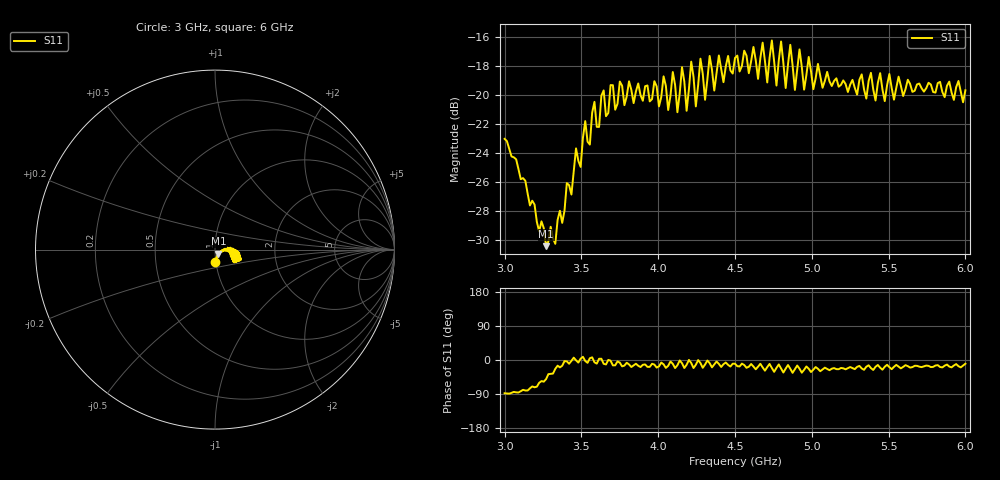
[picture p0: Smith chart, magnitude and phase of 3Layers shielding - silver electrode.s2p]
!  03/07/2025  15:49:02
! Ref Plane: 0.000 mm
# MHZ S MA R  50
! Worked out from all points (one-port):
!   201 points, 3 GHz to 6 GHz, reference 50 ohm
!   lowest |S11| = -30.4 dB at 3.27 GHz (marker M1), VSWR 1.06, Z = 51.9 - j2.41 ohm
!   |S11| at or under -10 dB: start of sweep to end of sweep
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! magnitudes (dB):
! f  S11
! 3 GHz  -23.0
! 3.27 GHz  -30.4
! 3.375 GHz  -28.8
! 3.525 GHz  -21.8
! 3.555 GHz  -23.4
! 3.585 GHz  -20.5
! 3.615 GHz  -22.2
! 3.645 GHz  -19.7
! 3.75 GHz  -19.1
! 4.005 GHz  -20.8
! 4.035 GHz  -18.7
! 4.065 GHz  -21.0
! 4.095 GHz  -18.4
! 4.125 GHz  -21.2
! 4.155 GHz  -18.1
! 4.185 GHz  -21.1
! 4.215 GHz  -17.7
! 4.245 GHz  -20.8
! 4.275 GHz  -17.5
! 4.305 GHz  -20.3
! 4.335 GHz  -17.3
! 4.365 GHz  -19.7
! 4.395 GHz  -17.3
! 4.5 GHz  -17.4
! 4.875 GHz  -18.0
! 5.25 GHz  -19.3
! 5.625 GHz  -18.9
! 6 GHz  -19.7
